| IBIS file stm32wba55_ufqfpn48-smps.ibs
[IBIS ver] 4.2
[File name] stm32wba55_ufqfpn48-smps.ibs
[File Rev] 1.2
[Date] 22-05-2024
[Source] Data Created at STMicroelectronics
[Notes]  File originated from ELDO simulations.
[Disclaimer]  This information is for modeling purpose only and is
   not guaranteed. The information is subject to change without
   notice.
[Copyright] Copyright 2024 STMicroelectronics Inc.
|   Component stm32wba55_ufqfpn48-smps
[Component] stm32wba55_ufqfpn48-smps
[Manufacturer] STMicroelectronics
[Package]
| variable   typ   min   max
R_pkg  0  NA  NA
L_pkg  0  NA  NA
C_pkg  0  NA  NA
[Pin]   signal_name   model_name
0  VSS  gnd
1  VSSSMPS  nc
2  VDDSMPS  nc
3  VLXSMPS  nc
4  PB12  io8_ft_100m_v33
5  PA8  io8_ft_100m_v33
6  PA7  io8_ft_100m_i2c_v33
7  PA6  io8_ft_100m_i2c_v33
8  VDDA  nc
9  PA5  io8_ft_100m_v33
10  PA2  io8_ft_100m_v33
11  VDD  power
12  PA1  io8_ft_100m_v33
13  PA0  io8_ft_100m_v33
14  PB9  io8_ft_100m_v33
15  PB8  io8_ft_100m_v33
16  PC15-OSC32_OUT  io8_ft_100m_tamp
17  PC14-OSC32_IN  io8_ft_100m_tamp
18  PC13  io8_ft_100m_v33
19  PB7  io8_ft_100m_v33
20  PB6  io8_ft_100m_v33
21  PB5  io8_ft_100m_v33
22  VDD  power
23  PB4  io8_ft_100m_v33
24  PB3  io8_ft_100m_i2c_v33
25  PA15  io8_ft_100m_i2c_v33
26  PA14  io8_ft_100m_v33
27  PA13  io8_ft_100m_v33
28  PA12  io8_ft_100m_v33
29  PA11  io8_ft_100m_v33
30  PB2  io8_ft_100m_i2c_v33
31  PB1  io8_ft_100m_i2c_v33
32  PB0  io8_ft_100m_v33
33  PB15  io8_ft_100m_v33
34  PH3-BOOT0  io8_ft_100m_v33
35  VDD  power
36  NRST  ioreset_v33
37  RF  nc
38  VDDHPA  nc
39  VDDANA  nc
40  VDDRF  nc
41  OSC_OUT  nc
42  OSC_IN  nc
43  VDDRFPA  nc
44  VDD  nc
45  VDD11  nc
46  PA10  io8_ft_100m_v33
47  PA9  io8_ft_100m_v33
48  PB14  io8_ft_100m_v33
[Package Model]   492-ufqfpn-7x7-48-smps-240513
[Pin Mapping]   pulldown_ref   pullup_ref   | Comment
0  gndio  nc
1  nc  nc
2  nc  nc
3  nc  nc
4  gndio  vddiom
5  gndio  vddiom
6  gndio  vddiom
7  gndio  vddiom
8  nc  nc
9  gndio  vddiom
10  gndio  vddiom
11  nc  vddiom
12  gndio  vddiom
13  gndio  vddiom
14  gndio  vddiom
15  gndio  vddiom
16  gndio  vddiom
17  gndio  vddiom
18  gndio  vddiom
19  gndio  vddiom
20  gndio  vddiom
21  gndio  vddiom
22  nc  vddiom
23  gndio  vddiom
24  gndio  vddiom
25  gndio  vddiom
26  gndio  vddiom
27  gndio  vddiom
28  gndio  vddiom
29  gndio  vddiom
30  gndio  vddiom
31  gndio  vddiom
32  gndio  vddiom
33  gndio  vddiom
34  gndio  vddiom
35  nc  vddiom
36  gndio  vddiom
37  nc  nc
38  nc  nc
39  nc  nc
40  nc  nc
41  nc  nc
42  nc  nc
43  nc  nc
44  nc  nc
45  nc  nc
46  gndio  vddiom
47  gndio  vddiom
48  gndio  vddiom
[Model Selector] io8_ft_100m_i2c_v33
io8_ft_100m_v33_ls_1v2  "GPIO_V33 100MHz - 5V tolerant - low speed - 1.2V range"
io8_ft_100m_v33_ls_1v8  "GPIO_V33 100MHz - 5V tolerant - low speed - 1.8V range"
io8_ft_100m_v33_ls_3v3  "GPIO_V33 100MHz - 5V tolerant - low speed - 3.3V range"
io8_ft_100m_v33_ms_1v2  "GPIO_V33 100MHz - 5V tolerant - med speed - 1.2V range"
io8_ft_100m_v33_ms_1v8  "GPIO_V33 100MHz - 5V tolerant - med speed - 1.8V range"
io8_ft_100m_v33_ms_3v3  "GPIO_V33 100MHz - 5V tolerant - med speed - 3.3V range"
io8_ft_100m_v33_fs_1v2  "GPIO_V33 100MHz - 5V tolerant - fast speed - 1.2V range"
io8_ft_100m_v33_fs_1v8  "GPIO_V33 100MHz - 5V tolerant - fast speed - 1.8V range"
io8_ft_100m_v33_fs_3v3  "GPIO_V33 100MHz - 5V tolerant - fast speed - 3.3V range"
io8_ft_100m_v33_hs_1v2  "GPIO_V33 100MHz - 5V tolerant - high speed - 1.2V range"
io8_ft_100m_v33_hs_1v8  "GPIO_V33 100MHz - 5V tolerant - high speed - 1.8V range"
io8_ft_100m_v33_hs_3v3  "GPIO_V33 100MHz - 5V tolerant - high speed - 3.3V range"
io8_ft_100m_i2c_v33_ls_1v2  "GPIO_V33 100MHz with I2C open-drain - 5V tolerant - low speed - 1.2V range"
io8_ft_100m_i2c_v33_ls_1v8  "GPIO_V33 100MHz with I2C open-drain - 5V tolerant - low speed - 1.8V range"
io8_ft_100m_i2c_v33_ls_3v3  "GPIO_V33 100MHz with I2C open-drain - 5V tolerant - low speed - 3.3V range"
io8_ft_100m_i2c_v33_ms_1v2  "GPIO_V33 100MHz with I2C open-drain - 5V tolerant - med speed - 1.2V range"
io8_ft_100m_i2c_v33_ms_1v8  "GPIO_V33 100MHz with I2C open-drain - 5V tolerant - med speed - 1.8V range"
io8_ft_100m_i2c_v33_ms_3v3  "GPIO_V33 100MHz with I2C open-drain - 5V tolerant - med speed - 3.3V range"
io8_ft_100m_i2c_v33_fs_1v2  "GPIO_V33 100MHz with I2C open-drain - 5V tolerant - fast speed - 1.2V range"
io8_ft_100m_i2c_v33_fs_1v8  "GPIO_V33 100MHz with I2C open-drain - 5V tolerant - fast speed - 1.8V range"
io8_ft_100m_i2c_v33_fs_3v3  "GPIO_V33 100MHz with I2C open-drain - 5V tolerant - fast speed - 3.3V range"
io8_ft_100m_i2c_v33_hs_1v2  "GPIO_V33 100MHz with I2C open-drain - 5V tolerant - high speed - 1.2V range"
io8_ft_100m_i2c_v33_hs_1v8  "GPIO_V33 100MHz with I2C open-drain - 5V tolerant - high speed - 1.8V range"
io8_ft_100m_i2c_v33_hs_3v3  "GPIO_V33 100MHz with I2C open-drain - 5V tolerant - high speed - 3.3V range"
io8_ft_100m_i2c_fmp_v33_3v3  "GPIO_V33 100MHz with I2C fm+ open-drain - 5V tolerant - low speed - 3.3V range"
[Model Selector] io8_ft_100m_tamp
io8_ft_100m_ls_1v2 "GPIO SPI - 5V tolerant - low speed - 1.2V range"
io8_ft_100m_ls_1v8 "GPIO SPI - 5V tolerant - low speed - 1.8V range"
io8_ft_100m_ls_3v3 "GPIO SPI - 5V tolerant - low speed - 3.3V range"
io8_ft_100m_ms_1v2 "GPIO SPI - 5V tolerant - med speed - 1.2V range"
io8_ft_100m_ms_1v8 "GPIO SPI - 5V tolerant - med speed - 1.8V range"
io8_ft_100m_ms_3v3 "GPIO SPI - 5V tolerant - med speed - 3.3V range"
io8_ft_100m_fs_1v2 "GPIO SPI - 5V tolerant - fast speed - 1.2V range"
io8_ft_100m_fs_1v8 "GPIO SPI - 5V tolerant - fast speed - 1.8V range"
io8_ft_100m_fs_3v3 "GPIO SPI - 5V tolerant - fast speed - 3.3V range"
io8_ft_100m_hs_1v2 "GPIO SPI - 5V tolerant - high speed - 1.2V range"
io8_ft_100m_hs_1v8 "GPIO SPI - 5V tolerant - high speed - 1.8V range"
io8_ft_100m_hs_3v3 "GPIO SPI - 5V tolerant - high speed - 3.3V range"
io8_ft_tamp_ls_1v2 "IO TAMPER_3V - 5V tolerant - low speed - 1.2V range"
io8_ft_tamp_ls_1v8 "IO TAMPER_3V - 5V tolerant - low speed - 1.8V range"
io8_ft_tamp_ls_3v3 "IO TAMPER_3V-  5V tolerant - low speed - 3.3V range"
io8_ft_tamp_ms_1v2 "IO TAMPER_3V - 5V tolerant - med speed - 1.2V range"
io8_ft_tamp_ms_1v8 "IO TAMPER_3V - 5V tolerant - med speed - 1.8V range"
io8_ft_tamp_ms_3v3 "IO TAMPER_3V - 5V tolerant - med speed - 3.3V range"
io8_ft_tamp_fs_1v2 "IO TAMPER_3V - 5V tolerant - fast speed - 1.2V range"
io8_ft_tamp_fs_1v8 "IO TAMPER_3V - 5V tolerant - fast speed - 1.8V range"
io8_ft_tamp_fs_3v3 "IO TAMPER_3V - 5V tolerant - fast speed - 3.3V range"
io8_ft_tamp_hs_1v2 "IO TAMPER_3V - 5V tolerant - high speed - 1.2V range"
io8_ft_tamp_hs_1v8 "IO TAMPER_3V - 5V tolerant - high speed - 1.8V range"
io8_ft_tamp_hs_3v3 "IO TAMPER_3V - 5V tolerant - high speed - 3.3V range"
[Model Selector] io8_ft_100m_v33
io8_ft_100m_v33_ls_1v2  "GPIO_V33 100MHz - 5V tolerant - low speed - 1.2V range"
io8_ft_100m_v33_ls_1v8  "GPIO_V33 100MHz - 5V tolerant - low speed - 1.8V range"
io8_ft_100m_v33_ls_3v3  "GPIO_V33 100MHz - 5V tolerant - low speed - 3.3V range"
io8_ft_100m_v33_ms_1v2  "GPIO_V33 100MHz - 5V tolerant - med speed - 1.2V range"
io8_ft_100m_v33_ms_1v8  "GPIO_V33 100MHz - 5V tolerant - med speed - 1.8V range"
io8_ft_100m_v33_ms_3v3  "GPIO_V33 100MHz - 5V tolerant - med speed - 3.3V range"
io8_ft_100m_v33_fs_1v2  "GPIO_V33 100MHz - 5V tolerant - fast speed - 1.2V range"
io8_ft_100m_v33_fs_1v8  "GPIO_V33 100MHz - 5V tolerant - fast speed - 1.8V range"
io8_ft_100m_v33_fs_3v3  "GPIO_V33 100MHz - 5V tolerant - fast speed - 3.3V range"
io8_ft_100m_v33_hs_1v2  "GPIO_V33 100MHz - 5V tolerant - high speed - 1.2V range"
io8_ft_100m_v33_hs_1v8  "GPIO_V33 100MHz - 5V tolerant - high speed - 1.8V range"
io8_ft_100m_v33_hs_3v3  "GPIO_V33 100MHz - 5V tolerant - high speed - 3.3V range"
[Model Selector] ioreset_v33
ioreset_v33_1v2 "Reset PAD. 5V tolerant. 1.2V range"
ioreset_v33_1v8 "Reset PAD. 5V tolerant. 1.8V range"
ioreset_v33_3v3 "Reset PAD. 5V tolerant. 3.3V range"
[Define Package Model]  492-ufqfpn-7x7-48-smps-240513
[Manufacturer]  Unknown
[OEM]  Unknown
[Description]  None
[Number Of Pins]  49
[Pin Numbers]
| Pin Num   Terminal Name
37 | RF
36 | NRST
13 | PA0
46 | PA10
29 | PA11
28 | PA12
27 | PA13
26 | PA14
25 | PA15
12 | PA1
10 | PA2
9 | PA5
7 | PA6
6 | PA7
5 | PA8
47 | PA9
32 | PB0
4 | PB12
48 | PB14
33 | PB15
31 | PB1
30 | PB2
24 | PB3
23 | PB4
21 | PB5
20 | PB6
19 | PB7
15 | PB8
14 | PB9
18 | PC13
17 | PC14-OSC32_IN
16 | PC15-OSC32_OUT
34 | PH3-BOOT0
45 | VDD11
40 | VDDRF
39 | VDDANA
11 | VDD
22 | VDD
8 | VDDA
44 | VDD
38 | VDDHPA
43 | VDDRFPA
2 | VDDSMPS
35 | VDD
3 | VLXSMPS
0 | VSS
1 | VSSSMPS
42 | OSC_IN
41 | OSC_OUT
[Model Data]
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[End Model Data]
[End Package Model]
|End [Component]
| Models and submodels in the file (52): io8_ft_100m_fs_1v2 (I/O), io8_ft_100m_fs_1v8 (I/O), io8_ft_100m_fs_3v3 (I/O), io8_ft_100m_hs_1v2 (I/O), io8_ft_100m_hs_1v8 (I/O), io8_ft_100m_hs_3v3 (I/O), io8_ft_100m_i2c_fmp_v33_3v3 (I/O_open_drain), io8_ft_100m_i2c_v33_fs_1v2 (I/O_open_drain), io8_ft_100m_i2c_v33_fs_1v8 (I/O_open_drain), io8_ft_100m_i2c_v33_fs_3v3 (I/O_open_drain), io8_ft_100m_i2c_v33_hs_1v2 (I/O_open_drain), io8_ft_100m_i2c_v33_hs_1v8 (I/O_open_drain), io8_ft_100m_i2c_v33_hs_3v3 (I/O_open_drain), io8_ft_100m_i2c_v33_ls_1v2 (I/O_open_drain), io8_ft_100m_i2c_v33_ls_1v8 (I/O_open_drain), io8_ft_100m_i2c_v33_ls_3v3 (I/O_open_drain), io8_ft_100m_i2c_v33_ms_1v2 (I/O_open_drain), io8_ft_100m_i2c_v33_ms_1v8 (I/O_open_drain), io8_ft_100m_i2c_v33_ms_3v3 (I/O_open_drain), io8_ft_100m_ls_1v2 (I/O), io8_ft_100m_ls_1v8 (I/O), io8_ft_100m_ls_3v3 (I/O), io8_ft_100m_ms_1v2 (I/O), io8_ft_100m_ms_1v8 (I/O), io8_ft_100m_ms_3v3 (I/O), io8_ft_100m_v33_fs_1v2 (I/O), io8_ft_100m_v33_fs_1v8 (I/O), io8_ft_100m_v33_fs_3v3 (I/O), io8_ft_100m_v33_hs_1v2 (I/O), io8_ft_100m_v33_hs_1v8 (I/O), io8_ft_100m_v33_hs_3v3 (I/O), io8_ft_100m_v33_ls_1v2 (I/O), io8_ft_100m_v33_ls_1v8 (I/O), io8_ft_100m_v33_ls_3v3 (I/O), io8_ft_100m_v33_ms_1v2 (I/O), io8_ft_100m_v33_ms_1v8 (I/O), io8_ft_100m_v33_ms_3v3 (I/O), io8_ft_tamp_fs_1v2 (I/O), io8_ft_tamp_fs_1v8 (I/O), io8_ft_tamp_fs_3v3 (I/O), io8_ft_tamp_hs_1v2 (I/O), io8_ft_tamp_hs_1v8 (I/O), io8_ft_tamp_hs_3v3 (I/O), io8_ft_tamp_ls_1v2 (I/O), io8_ft_tamp_ls_1v8 (I/O), io8_ft_tamp_ls_3v3 (I/O), io8_ft_tamp_ms_1v2 (I/O), io8_ft_tamp_ms_1v8 (I/O), io8_ft_tamp_ms_3v3 (I/O), ioreset_v33_1v2 (I/O_open_drain), ioreset_v33_1v8 (I/O_open_drain), ioreset_v33_3v3 (I/O_open_drain)
